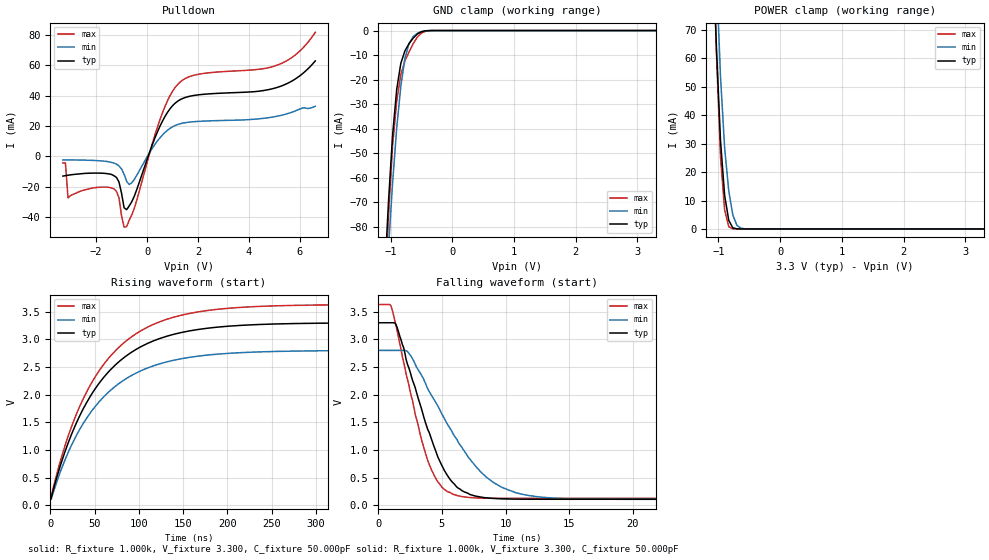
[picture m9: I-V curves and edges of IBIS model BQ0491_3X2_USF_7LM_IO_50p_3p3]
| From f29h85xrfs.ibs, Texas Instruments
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|   Model BQ0491_3X2_USF_7LM_IO_50p_3p3
[Model]   BQ0491_3X2_USF_7LM_IO_50p_3p3
Model_type   I/O_open_drain
Polarity   Non-Inverting
Enable   Active-Low
Vinl =   0.800V
Vinh =   2.000V
Vmeas =  1.650V
Cref =   50.000pF
Rref =   1.000k
Vref =   3.300V
|   typ   min   max
C_comp   1.084pF   1.003pF   1.123pF
[Model Spec]
Vinh   2.000V   2.000V   2.000V
Vinl   0.800V   0.800V   0.800V
[Temperature Range]   25   155   -40
[Voltage Range]   3.300V   2.800V   3.630V
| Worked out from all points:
|   slope of the pulldown table from 0 to 0.495 V, typ, clamps not added: 22.9 ohm
|   GND clamp passes 1 mA (typ) near -0.53 V on its own axis
|   POWER clamp passes 1 mA (typ) near -0.78 V on its own axis
|   rising waveform, R_fixture 1.000k, V_fixture 3.300, C_fixture 50.000pF: 20-80 % time 70.6ns typ, 70.6ns min, 70.6ns max; typ from 0.109 V to 3.3 V
|   falling waveform, R_fixture 1.000k, V_fixture 3.300, C_fixture 50.000pF: 20-80 % time 2.77ns typ, 4.28ns min, 2.18ns max; typ from 3.3 V to 0.109 V
[Pulldown]
|Voltage   I(typ)   I(min)   I(max)
-3.3V     -13.02mA   -2.341mA   -4.302mA
-3.2V     -12.73mA   -2.337mA   -4.378mA
-3.1V     -12.44mA   -2.348mA   -27.4mA
-1.3V     -12.73mA   -4.396mA   -21.37mA
-1.1V     -16.92mA   -6.309mA   -27.33mA
-900mV    -33.88mA   -11.82mA   -46.69mA
-800mV    -35.17mA   -16.44mA   -46.34mA
-600mV    -29.93mA   -17.47mA   -38.61mA
500mV     19.62mA    12.09mA    23.89mA
1.2V      36.37mA    21.01mA    47.41mA
5.1V      45.45mA    26.46mA    60.14mA
6.6V      62.95mA    33.05mA    81.82mA
[GND_clamp]
|Voltage   I(typ)   I(min)   I(max)
-3.3V     -1.477A    -1.275A    -1.767A
-1.1V     -102.3mA   -117.4mA   -113.6mA
-1.033V   -69.62mA   -88.44mA   -75.69mA
-967mV    -42.73mA   -62.13mA   -47.02mA
-900mV    -23.96mA   -39.74mA   -28.87mA
-833mV    -13.32mA   -22.64mA   -17.88mA
-767mV    -8.289mA   -11.35mA   -12.33mA
-700mV    -5.352mA   -5.293mA   -8.734mA
-567mV    -1.458mA   -1.135mA   -2.736mA
-433mV    -112.7uA   -134.1uA   -294.8uA
-300mV    -3.58uA    -9.04uA    -6.616uA
3.3V      0A         0A         0A
[POWER_clamp]
|Voltage   I(typ)   I(min)   I(max)
-3.3V     1.901A     2.191A     2.069A
-1.1V     105.6mA    134.8mA    109.4mA
-1.033V   63.91mA    89.93mA    62.06mA
-967mV    31.18mA    53.67mA    25.42mA
-900mV    11.84mA    28.57mA    6.708mA
-833mV    3.029mA    13.38mA    772.2uA
-767mV    401uA      4.887mA    44.81uA
-700mV    39.92uA    1.256mA    4.586uA
-633mV    5.005uA    258uA      1.414uA
-567mV    1.06uA     50.07uA    519.2nA
3.3V      0A         0A         0A
[Ramp]
| variable   typ   min   max
dV/dt_r   1.914/1.296n   1.615/1.263n   2.103/1.336n
dV/dt_f   1.914/0.125n   1.615/0.208n   2.103/98.310p
R_load = 1.000k
[Rising Waveform]
R_fixture= 1.000k
V_fixture= 3.300
V_fixture_min= 2.800
V_fixture_max= 3.630
C_fixture= 50.000pF
|time   V(typ)   V(min)   V(max)
0s        109.4mV    108.1mV    125.8mV
16.5ns    965.3mV    813.3mV    1.072V
31.6ns    1.563V     1.326V     1.728V
48.7ns    2.059V     1.746V     2.27V
68.7ns    2.463V     2.088V     2.712V
90.7ns    2.757V     2.338V     3.034V
116.7ns   2.974V     2.523V     3.273V
187.7ns   3.219V     2.731V     3.541V
369.7ns   3.298V     2.798V     3.628V
2us       3.3V       2.8V       3.63V
[Falling Waveform]
R_fixture= 1.000k
V_fixture= 3.300
V_fixture_min= 2.800
V_fixture_max= 3.630
C_fixture= 50.000pF
|time   V(typ)   V(min)   V(max)
0s        3.3V       2.8V       3.63V
1ns       3.3V       2.8V       3.606V
1.4ns     3.266V     2.8V       3.251V
2.3ns     2.549V     2.782V     2.275V
3.4ns     1.744V     2.352V     1.189V
4.6ns     928.6mV    1.829V     454.9mV
6.3ns     307.8mV    1.135V     170.9mV
9.4ns     120.3mV    365.3mV    126.4mV
26.1ns    109.3mV    108.1mV    125.7mV
2us       109.3mV    108.1mV    125.7mV
